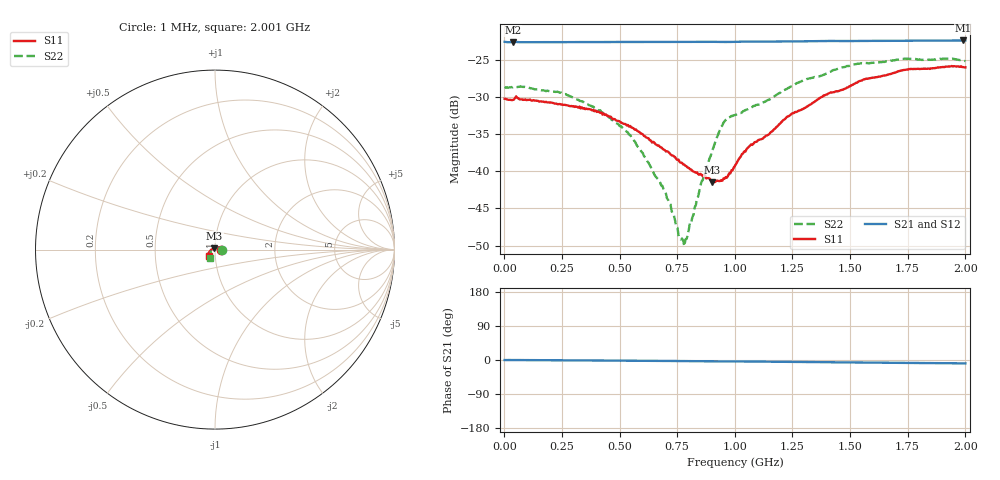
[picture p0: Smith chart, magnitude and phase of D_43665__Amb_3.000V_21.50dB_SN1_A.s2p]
! device id: 43665_
! dir: \\malibu\benchdata\1_engineers\tn_data\43665_75ohm\new\sparar\43665_\amb\3p000v\21p50db
! Serial: 1
! Insertion: A
! Temp: Amb
! VDD: 3.000V
! Attenuation Step: 21.50dB
! IDD: 1.449760e+00mA
! FILE NAME
! DATE 03-27-2009 08:38:37
! CORRECTED  DATA
#  Hz  S  RI  R  75
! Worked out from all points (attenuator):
!   401 points, 1 MHz to 2.001 GHz, reference 75 ohm
!   highest |S21| = -22.42 dB at 1.991 GHz (marker M1); lowest = -22.7 dB at 36 MHz (marker M2)
!   lowest |S11| = -41.5 dB at 901 MHz (marker M3), VSWR 1.02, Z = 74.5 + j1.14 ohm
!   |S11| at or under -10 dB: start of sweep to end of sweep
!   |S22| runs from -50.1 to -24.9 dB; largest |S21 - S12| = 0.00039
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1000000  0.0307 -0.000119  0.0741 -0.000164  0.0737 -0.000236  0.0368 -0.000385
3.6e7  0.0301 0.000929  0.0736 -0.00015  0.0736 -0.000106  0.0366 0.00102
2.36e8  0.0276 0.00599  0.0737 -0.000932  0.0738 -0.000914  0.033 0.00798
3.36e8  0.0256 0.00795  0.0738 -0.00143  0.0738 -0.00138  0.0276 0.0103
5.26e8  0.0178 0.0107  0.0739 -0.00235  0.0739 -0.00225  0.0161 0.00966
6.71e8  0.0101 0.0109  0.0739 -0.00304  0.0739 -0.00286  0.00577 0.00638
7.11e8  0.0081 0.0108  0.074 -0.00327  0.074 -0.00311  0.00334 0.00544
7.56e8  0.00556 0.0106  0.0741 -0.00353  0.0741 -0.0034  -0.000536 0.00367
7.81e8  0.0043 0.0102  0.0741 -0.00371  0.0741 -0.00358  -0.00236 0.00206
7.91e8  0.00363 0.0101  0.0741 -0.0038  0.0741 -0.00366  -0.00323 0.00136
8.56e8  -0.000301 0.00945  0.074 -0.00427  0.0741 -0.00413  -0.00758 -0.00387
9.01e8  -0.00347 0.00766  0.0739 -0.00464  0.074 -0.00443  -0.0112 -0.00784
9.51e8  -0.00621 0.00642  0.0737 -0.00476  0.0738 -0.00453  -0.0185 -0.0103
1.001e9  -0.00913 0.00592  0.0739 -0.00474  0.074 -0.00455  -0.0221 -0.00888
1.061e9  -0.014 0.00415  0.0742 -0.00527  0.0743 -0.00504  -0.0233 -0.0124
1.236e9  -0.0232 -0.00345  0.0743 -0.00637  0.0744 -0.00615  -0.0274 -0.024
1.336e9  -0.0274 -0.00799  0.0745 -0.00703  0.0747 -0.00675  -0.0299 -0.03
1.546e9  -0.0353 -0.0199  0.0746 -0.00868  0.0748 -0.00853  -0.0322 -0.0421
1.671e9  -0.0366 -0.0259  0.0746 -0.00956  0.0749 -0.00944  -0.0318 -0.0446
1.756e9  -0.0372 -0.0312  0.0747 -0.0101  0.075 -0.0101  -0.0308 -0.0478
1.991e9  -0.0326 -0.038  0.0748 -0.0116  0.0749 -0.0117  -0.0278 -0.0481
2.001e9  -0.0323 -0.038  0.0747 -0.0117  0.0749 -0.0117  -0.0274 -0.0476
